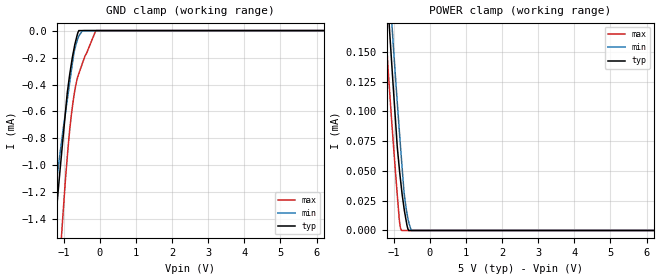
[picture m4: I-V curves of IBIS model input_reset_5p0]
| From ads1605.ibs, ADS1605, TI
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|   INPUT_RESET 5.0V Model
[Model]   input_reset_5p0
Model_type   Input
Vinl = 1.5
Vinh = 3.5
|   typ   min   max
|   (nom PVT)   (Fast PVT)   (Slow PVT)
C_comp   7.521e-13   7.338e-13   7.723e-13
|Where nom PVT is NOM Process, 5.0V,39C
|   Fast PVT is Strong Process, 5.25V, -40C
|   Slow PVT is Weak Process, 4.75V, 99C
[Model Spec]
Vinl   1.5   1.425   1.575
Vinh   3.5   3.325   3.675
[Voltage Range]   5   4.75   5.25
|Ambient Temperature   25   85   -40
|Junction Temperature
[Temperature Range]   39   99   -40
[Power Clamp Reference]   5   4.75   5.25
[GND Clamp Reference]   0   0   0
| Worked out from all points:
|   GND clamp passes 1 mA (typ) near -1.09 V on its own axis
|   POWER clamp passes 1 mA (typ) near -2.76 V on its own axis
[GND Clamp]
|   Voltage   I(typ)   I(min)   I(max)
-5V       -13.49mA   -9.525mA   -24.92mA
-1.414V   -1.982mA   -1.574mA   -3.397mA
-1.333V   -1.731mA   -1.397mA   -2.939mA
-1.27V    -1.537mA   -1.264mA   -2.585mA
-1.052V   -889.4uA   -805.1uA   -1.483mA
-905mV    -468.4uA   -518.4uA   -944.7uA
-836.7mV  -328.4uA   -388.4uA   -741.2uA
-710.7mV  -127.6uA   -157uA     -471.7uA
-582.5mV  0A         -40.95uA   -319.2uA
-487.5mV  0A         -2.458uA   -246.2uA
-112.3mV  0A         0A         0A
10V       0A         0A         0A
[POWER Clamp]
|   Voltage   I(typ)   I(min)   I(max)
-5V       2.166mA    2.195mA    2.125mA
-1.286V   250.1uA    286.1uA    199.6uA
-1.14V    179.2uA    216.1uA    128.1uA
-1.052V   138.2uA    174uA      89.62uA
-905mV    71.19uA    108.6uA    30.83uA
-842mV    50.81uA    82.48uA    7.686uA
-784.3mV  34.81uA    59.16uA    0A
-715.5mV  18.82uA    32.18uA    0A
-658.5mV  8.579uA    18.98uA    0A
-592mV    0A         7.789uA    0A
-501.8mV  0A         0A         0A
10V       0A         0A         0A
